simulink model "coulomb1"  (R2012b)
settings: Solver=ode45  StartTime=0.0  StopTime=10.0  RelTol=1e-3
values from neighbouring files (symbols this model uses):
  c = 2200    [coulomb_1.m]    (also in coulomb_10.m = 0.1; coulomb_11.m = 0; coulomb_2.m; coulomb_3.m)
  Fex_ampl = 800    [coulomb_1.m]    (also in coulomb_2.m; coulomb_3.m; coulomb_4.m; coulomb_5.m)
  FG = 500    [coulomb_1.m]    (also in coulomb_10.m = 10; coulomb_11.m = 10; coulomb_2.m; coulomb_3.m)
  fu = 0.02    [coulomb_1.m]    (also in coulomb_2.m; coulomb_3.m; coulomb_4.m; coulomb_5.m = 0.1)
  m = 400    [coulomb_1.m]    (also in coulomb_10.m = 10; coulomb_11.m = 10; coulomb_2.m; coulomb_3.m)
  v0 = 0    [coulomb_1.m]    (also in coulomb_2.m; coulomb_3.m; coulomb_4.m; coulomb_5.m)
  y0 = 0    [coulomb_1.m]    (also in coulomb_2.m; coulomb_3.m; coulomb_4.m; coulomb_5.m)

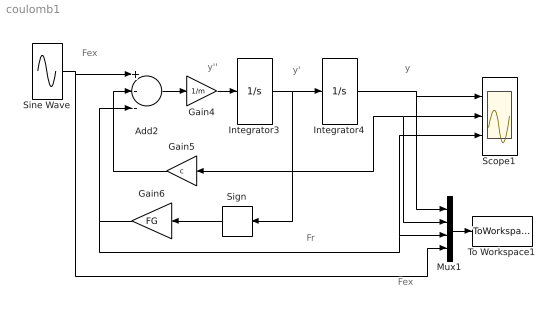
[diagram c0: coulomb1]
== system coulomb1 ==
  note: Fex
  note: Fr
  note: Fex
  note: y
  note: y'
  note: y''
  Add2 : Sum  Inputs=+--
  Gain4 : Gain  Gain=1/m
  Gain5 : Gain  Gain=c
  Gain6 : Gain  Gain=FG
  Integrator3 : Integrator  InitialCondition=v0
  Integrator4 : Integrator  InitialCondition=y0
  Mux1 : Mux
  Scope1 : Scope  NumInputPorts=3
  Sign : Signum  ZeroCross=off
  Sine Wave : Sin  Amplitude=Fex_ampl  Frequency=2*pi*fu  SampleTime=0
  To Workspace1 : ToWorkspace  VariableName=y  SampleTime=-1  SaveFormat=Structure With Time
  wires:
  Add2/1 -> Gain4/1
  Gain4/1 -> Integrator3/1
  Gain5/1 -> Add2/2
  Integrator4/1 -> Scope1/1, Mux1/1
  Integrator3/1 -> Scope1/2, Mux1/2, Gain5/1, Sign/1, Integrator4/1
  Gain6/1 -> Add2/3, Mux1/3, Scope1/3
  Mux1/1 -> To Workspace1/1
  Sign/1 -> Gain6/1
  Sine Wave/1 -> Mux1/4, Add2/1
